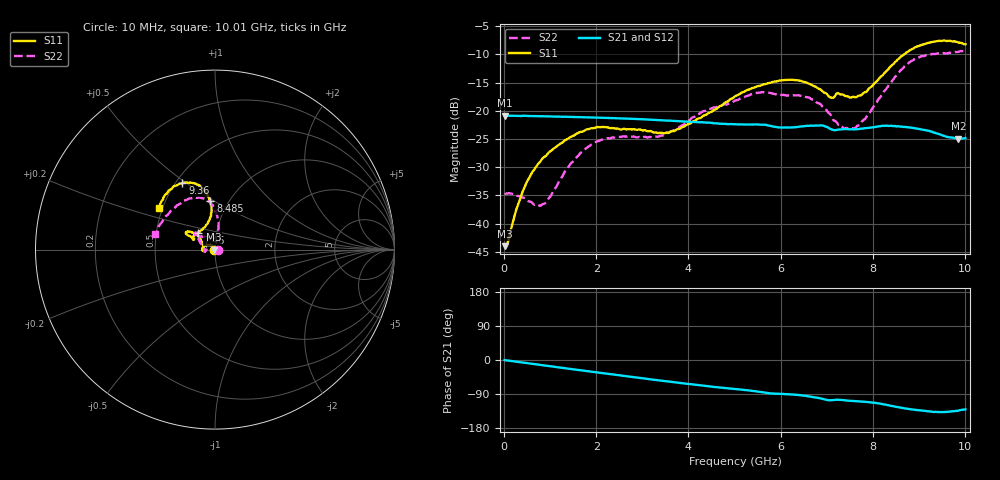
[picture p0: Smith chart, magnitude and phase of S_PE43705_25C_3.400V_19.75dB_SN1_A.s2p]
! Device ID: PE43705
! Serial: 1
! Insertion: A
! Impedance: 50 ohm
! Temp: 25C
! VDD: 3.400V
! Attenuation Step: 19.75dB
#  Hz  S  RI  R  50
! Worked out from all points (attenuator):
!   401 points, 10 MHz to 10.01 GHz, reference 50 ohm
!   highest |S21| = -20.83 dB at 10 MHz (marker M1); lowest = -25.0 dB at 9.86 GHz (marker M2)
!   lowest |S11| = -44.0 dB at 10 MHz (marker M3), VSWR 1.01, Z = 49.4 + j0.0445 ohm
!   |S11| at or under -10 dB: start of sweep to 8.678 GHz
!   |S22| runs from -36.8 to -9.3 dB; largest |S21 - S12| = 0.0011
!   S11 on the Smith chart (normalised r, x): 10 MHz: 0.99, +0.00; 7.46 GHz: 0.81, +0.16; 8.485 GHz: 0.82, +0.48; 9.36 GHz: 0.54, +0.48; 10.01 GHz: 0.48, +0.26
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1e7  -0.00631 0.000451  0.0908 -0.000322  0.091 -0.000351  0.0183 0.000254
8.5e7  -0.00602 0.0035  0.0905 -0.00241  0.0905 -0.00238  0.0185 0.00197
4.1e8  -0.0105 0.0166  0.09 -0.0105  0.0897 -0.0109  0.0134 0.0105
6.35e8  -0.0184 0.023  0.0883 -0.0166  0.0884 -0.0165  0.00549 0.0138
9.1e8  -0.0303 0.0262  0.0864 -0.0234  0.0864 -0.0233  -0.00674 0.0139
1.685e9  -0.0633 0.0157  0.0779 -0.0406  0.0779 -0.0406  -0.0433 0.000673
2.235e9  -0.0716 -7.68e-05  0.0697 -0.0513  0.0697 -0.0511  -0.0561 -0.011
3.36e9  -0.0636 0.00213  0.0488 -0.0667  0.0489 -0.0667  -0.0592 0.00303
3.86e9  -0.0669 0.0249  0.0389 -0.0706  0.0389 -0.0706  -0.0708 0.0233
5.01e9  -0.1043 0.0849  0.0177 -0.0739  0.0177 -0.074  -0.0983 0.0744
5.535e9  -0.1343 0.0977  0.00803 -0.0752  0.00819 -0.0752  -0.1117 0.0919
6.01e9  -0.1575 0.0991  0.000873 -0.0712  0.000985 -0.0713  -0.1054 0.0897
6.685e9  -0.1492 0.0786  -0.00968 -0.0731  -0.00955 -0.0732  -0.0987 0.0781
7.085e9  -0.116 0.0617  -0.0191 -0.0665  -0.0192 -0.0664  -0.059 0.0711
7.46e9  -0.0951 0.0948  -0.0204 -0.0658  -0.0201 -0.0655  -0.02 0.0665
7.76e9  -0.0545 0.1275  -0.0234 -0.0655  -0.0231 -0.0656  0.00501 0.0797
8.36e9  -0.0191 0.24  -0.0367 -0.0637  -0.0366 -0.0642  0.0163 0.1715
8.485e9  -0.0258 0.2696  -0.0401 -0.0615  -0.0396 -0.0618  0.0081 0.2002
8.885e9  -0.0787 0.3486  -0.0462 -0.0533  -0.0458 -0.0531  -0.0511 0.2781
9.36e9  -0.1814 0.3695  -0.0465 -0.0434  -0.0467 -0.0433  -0.1616 0.2753
9.86e9  -0.2891 0.2786  -0.0389 -0.041  -0.0388 -0.0408  -0.297 0.1517
1.001e10  -0.3136 0.2309  -0.0371 -0.0438  -0.0374 -0.0441  -0.3326 0.0871
